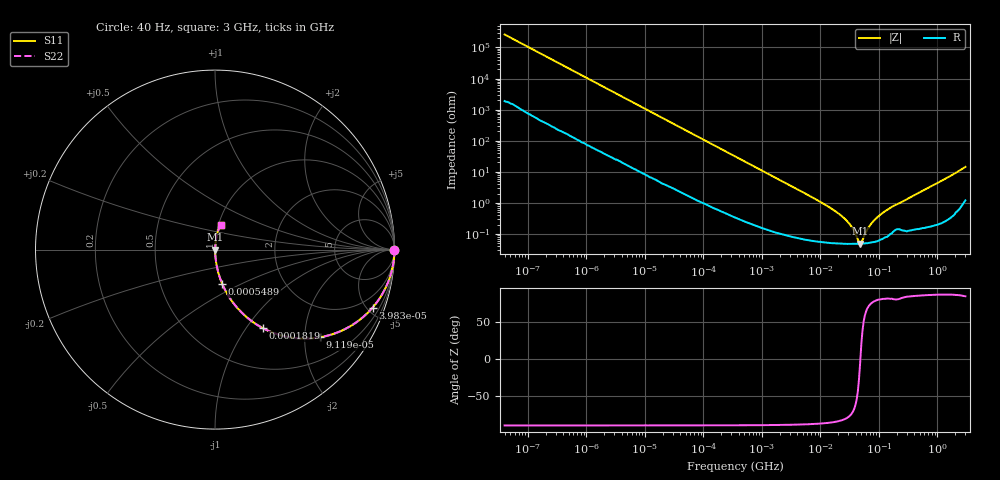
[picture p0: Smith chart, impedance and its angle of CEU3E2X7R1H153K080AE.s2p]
! S-parameter Generated by TDK Corporation
! Copyright(C) 2015 TDK Corporation.
! All Rights Reserved.
! TDK P/N: CEU3E2X7R1H153K080AE (Multilayer Ceramic Chip Capacitors)
! Property: C=15nF
! Size(LxWxT): 1.6x0.8x0.8mm, 0.063x0.031x0.031inches
! Model Type: s2p (Touchstone File Format Version 1.0)
! Frequency: DC=Yes Start=0.00004MHz Stop=3000MHz 396points Log-sweep
! Note: This model was converted from impedance.
! Model Generated on Jun. 23, 2015
! Hash(MD5):
! Port Assignments:
!  1 ---| |--- 2
! Applicable Conditions:
!  Temperature = 25 degC
!  DC Bias Voltage = 0 V
!  Small Signal Operation
! Terms and conditions regarding TDK Simulation Models
! (1)This simulation model is being provided solely for informational purposes. Please refer to the specifications of the products in terms of detailed characteristics of such products.
! (2)In no event shall TDK Corporation of any of its subsidiaries be liable for any loss or damage arising, directly or indirectly,
!  From any information contained in this simulation model, including, but not limited to loss or damages arising from any inaccuracies, omissions or errors in connection with such information.
! (3)Any and all copyrights on this simulation model are owned by TDK Corporation.
!  Duplication or redistribution of this simulation model without prior written permission from TDK Corporation is prohibited.
! (4)This simulation model is subject to any modification or change without any prior notice.
! (5)Neither TDK Corporation nor any of its subsidiaries shall make any warranty, express or implied,
!  Including but not limited to the correctness, implied warranties of merchantability and fitness for a particular purpose with respect to this simulation models.
! (6)The use of this simulation model shall be deemed to have consented to the terms and conditions hereof.
# MHz S MA R 50
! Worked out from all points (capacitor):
!   395 points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, 40 Hz to 3 GHz, reference 50 ohm
!   read as one part in series: C = 15.2 nF near 41.88 Hz
!   lowest |Z| = 49.2 mohm at 47.67 MHz (marker M1)
!   series resonance near 48.1 MHz, so ESL is about 720 pH
!   S11 on the Smith chart (normalised r, x): 40 Hz: open; 39.83 kHz: 1.04, -5.43; 91.19 kHz: 1.02, -2.38; 181.9 kHz: 1.01, -1.20; 548.9 kHz: 1.00, -0.40; 3 GHz: 1.02, +0.29
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4e-05  1 -0.0  0.0003815 89.6  0.0003815 89.6  1 -0.0
0.000834128  0.9999 -0.5  0.007862 89.2  0.007862 89.2  0.9999 -0.5
0.005256919  0.9984 -2.8  0.04903 86.8  0.04903 86.8  0.9984 -2.8
0.01739424  0.986 -9.2  0.1593 80.4  0.1593 80.4  0.986 -9.2
0.0398272  0.9358 -20.2  0.3448 69.4  0.3448 69.4  0.9358 -20.2
0.09119145  0.7625 -39.8  0.6403 49.7  0.6403 49.7  0.7625 -39.8
0.1818721  0.5119 -58.7  0.8541 30.8  0.8541 30.8  0.5119 -58.7
0.3464102  0.3004 -71.9  0.9506 17.5  0.9506 17.5  0.3004 -71.9
0.5488647  0.1957 -78.0  0.9783 11.3  0.9783 11.3  0.1957 -78.0
1.581893  0.06965 -85.1  0.9964 4.0  0.9964 4.0  0.06965 -85.1
7.22376  0.01515 -86.9  0.9993 0.9  0.9993 0.9  0.01515 -86.9
15.79611  0.006371 -85.1  0.9995 0.4  0.9995 0.4  0.006371 -85.1
26.2067  0.003061 -80.8  0.9995 0.2  0.9995 0.2  0.003061 -80.8
34.54118  0.001653 -73.0  0.9995 0.1  0.9995 0.1  0.001653 -73.0
47.67047  0.0004917 -4.9  0.9995 0.0  0.9995 0.0  0.0004917 -4.9
49.91566  0.0005267 19.9  0.9995 -0.0  0.9995 -0.0  0.0005267 19.9
62.83103  0.001371 68.4  0.9995 -0.1  0.9995 -0.1  0.001371 68.4
75.53079  0.002263 76.2  0.9995 -0.1  0.9995 -0.1  0.002263 76.2
104.2405  0.004094 80.7  0.9993 -0.2  0.9993 -0.2  0.004094 80.7
150.6385  0.006665 81.6  0.999 -0.4  0.999 -0.4  0.006665 81.6
1040.901  0.04545 84.8  0.9969 -2.6  0.9969 -2.6  0.04545 84.8
3000  0.1412 77.1  0.9782 -8.1  0.9782 -8.1  0.1412 77.1
